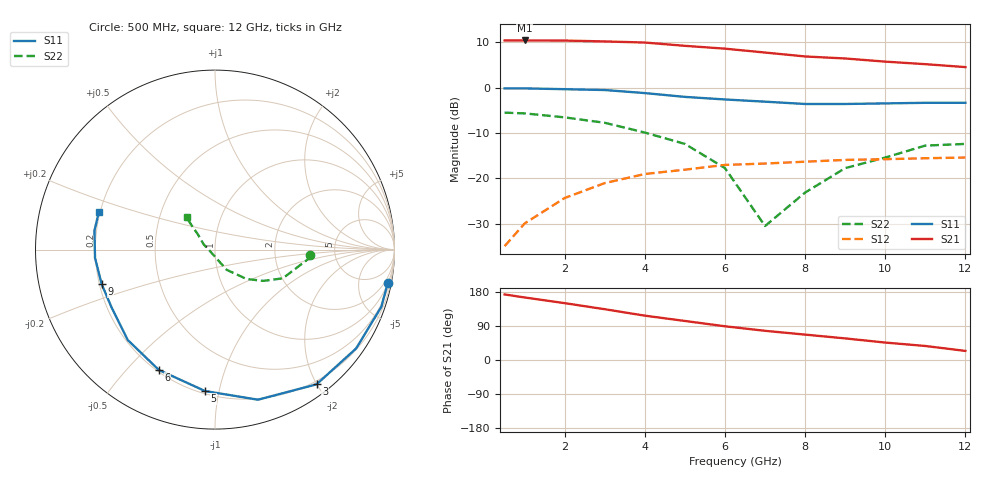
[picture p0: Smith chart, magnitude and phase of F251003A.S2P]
!ATF-25100
!S-PARAMETERS at Vds=3V  Id=20mA.  LAST UPDATED 07-22-92
# ghz s ma r 50
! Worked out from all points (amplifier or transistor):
!   13 points, 500 MHz to 12 GHz, reference 50 ohm
!   highest |S21| = 10.4 dB at 1 GHz (marker M1)
!   |S21| within 3 dB of that: start of sweep to 7.396 GHz
!   unconditionally stable (mu >= 1): 7.944 GHz to end of sweep
!   at 2 GHz: K = 0.24, MSG = 17.3 dB, |S12| = -24.3 dB
!   at 6 GHz: K = 0.73, MSG = 12.8 dB, |S12| = -17.0 dB
!   at 12 GHz: K = 1.06, MAG = 8.4 dB, |S12| = -15.4 dB
!   lowest NFmin = 0.50 dB at 500 MHz
!   S11 on the Smith chart (normalised r, x): 500 MHz: 1, -10; 3 GHz: 0.15, -2.00; 5 GHz: 0.22, -0.91; 6 GHz: 0.21, -0.62; 9 GHz: 0.21, -0.14; 12 GHz: 0.20, +0.15
0.5  0.98 -11.0  3.3 173.0  0.018 89.0  0.53 -3.0
1  0.98 -19.0  3.3 165.0  0.032 84.0  0.52 -6.0
2  0.96 -35.0  3.29 150.0  0.061 74.0  0.47 -12.0
3  0.94 -53.0  3.22 134.0  0.089 64.0  0.41 -23.0
4  0.87 -74.0  3.13 117.0  0.112 55.0  0.32 -33.0
5  0.79 -94.0  2.88 103.0  0.125 49.0  0.24 -43.0
6  0.74 -115.0  2.68 89.0  0.141 39.0  0.13 -60.0
7  0.7 -134.0  2.43 77.0  0.146 35.0  0.03 -167.0
8  0.66 -151.0  2.2 67.0  0.153 32.0  0.07 155.0
9  0.66 -163.0  2.09 57.0  0.16 25.0  0.13 138.0
10  0.67 -176.0  1.93 46.0  0.163 23.0  0.17 135.0
11  0.68 171.0  1.81 37.0  0.167 18.0  0.23 132.0
12  0.68 162.0  1.68 24.0  0.17 9.0  0.24 130.0
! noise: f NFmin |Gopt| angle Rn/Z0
0.5  0.5  0.96  5  1.15
1  0.5  0.91  11  1.03
2  0.6  0.83  22  0.79
4  0.8  0.57  63  0.67
6  1  0.5  101  0.23
8  1.2  0.47  135  0.34
